PROGRAM MAIN_CM

VAR CONSTANT
	cInitRms			: ST_CM_RMS_InitPars := (nChannels:= 1,
												 nBufferLength:= cRMSBuffer, 
												 fDecibelThreshold:= cCM_MinArgLog10, 
												 bTransformToDecibel:= FALSE);
END_VAR

VAR
	fbRms				: FB_CMA_RMS := (stInitPars := cInitRms, 
										 nOwnID:= eID_RMS, aDestIDs:= [eID_Sink]);	

	fbErrHist			: FB_HRErrHist; // error monitoring	
	
END_VAR

fbRms.Call();
IF fbRms.bError THEN
	fbErrHist.AddError(bErr:=TRUE, hrErrCode:=fbRms.hrErrorCode, sErrSource:='MAIN_CM.fbRms.call'); // error monitoring
	// ToDo: if error
END_IF

END_PROGRAM
